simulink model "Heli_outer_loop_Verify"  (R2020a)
settings: Solver=FixedStepDiscrete  StartTime=0.0  StopTime=10.0  FixedStep=0.01  RelTol=1e-3
undefined symbols (not defined in the file or in its folder): sldvsubsys
libraries: sldvlib x3

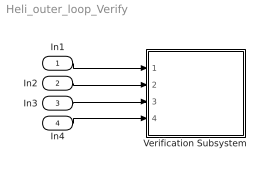
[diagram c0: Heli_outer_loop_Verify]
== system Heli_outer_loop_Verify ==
  In1 : Inport
  In2 : Inport  Port=2
  In3 : Inport  Port=3
  In4 : Inport  Port=4
  Verification Subsystem : Subsystem  Tag=VerificationSubsystem  DisableCoverage=on  LoadFcn=sldvsubsys('check')  TreatAsAtomicUnit=on  SimViewingDevice=on  mask(VerificationSubsystem){}
      mask init:
      | sldvsubsys('maskInit');
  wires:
  In1/1 -> Verification Subsystem/1(In1)
  In2/1 -> Verification Subsystem/2(In2)
  In3/1 -> Verification Subsystem/3(In3)
  In4/1 -> Verification Subsystem/4(In4)

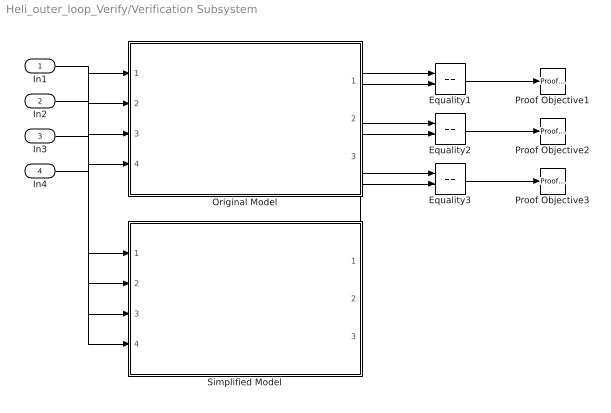
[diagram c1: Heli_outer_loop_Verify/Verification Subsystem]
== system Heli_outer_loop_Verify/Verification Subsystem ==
  In1 : Inport
  In2 : Inport  Port=2
  In3 : Inport  Port=3
  In4 : Inport  Port=4
  Equality1 : RelationalOperator  Operator===  OutDataTypeStr=boolean  RndMeth=Simplest
  Equality2 : RelationalOperator  Operator===  OutDataTypeStr=boolean  RndMeth=Simplest
  Equality3 : RelationalOperator  Operator===  OutDataTypeStr=boolean  RndMeth=Simplest
  Original Model : ModelReference  ModelNameDialog=Heli_outer_loop_Original  SimulationMode=Normal  ModelReferenceVersion=1.79
  Proof Objective1 : sldvlib/Objectives and Constraints/Proof Objective  enabled=on  customAVTBlockType=Proof Objective  intervals=true  dispValues=on  outEnabled=off  enableStopSim=off
  Proof Objective2 : sldvlib/Objectives and Constraints/Proof Objective  enabled=on  customAVTBlockType=Proof Objective  intervals=true  dispValues=on  outEnabled=off  enableStopSim=off
  Proof Objective3 : sldvlib/Objectives and Constraints/Proof Objective  enabled=on  customAVTBlockType=Proof Objective  intervals=true  dispValues=on  outEnabled=off  enableStopSim=off
  Simplified Model : ModelReference  ModelNameDialog=Heli_outer_loop_New  SimulationMode=Normal  ModelReferenceVersion=1.84
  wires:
  In1/1 -> Original Model/1, Simplified Model/1
  In2/1 -> Original Model/2, Simplified Model/2
  In3/1 -> Original Model/3, Simplified Model/3
  In4/1 -> Original Model/4, Simplified Model/4
  Original Model/1 -> Equality1/1
  Simplified Model/1 -> Equality1/2
  Equality1/1 -> Proof Objective1/1
  Original Model/2 -> Equality2/1
  Simplified Model/2 -> Equality2/2
  Equality2/1 -> Proof Objective2/1
  Original Model/3 -> Equality3/1
  Simplified Model/3 -> Equality3/2
  Equality3/1 -> Proof Objective3/1
